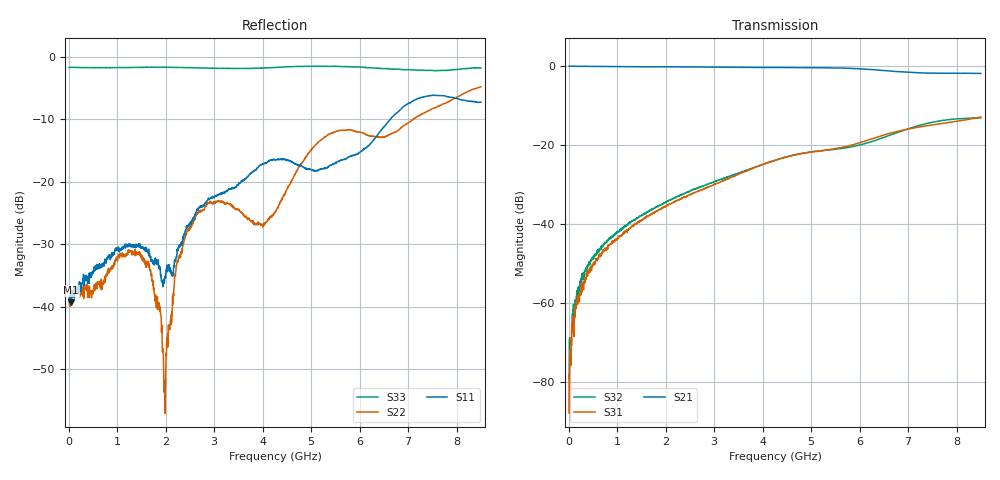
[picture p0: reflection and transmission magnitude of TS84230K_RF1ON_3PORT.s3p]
! Created with skrf (http://scikit-rf.org).
# Hz S RI R 50.0
!freq ReS11 ImS11 ReS12 ImS12 ReS13 ImS13
! ReS21 ImS21 ReS22 ImS22 ReS23 ImS23
! ReS31 ImS31 ReS32 ImS32 ReS33 ImS33
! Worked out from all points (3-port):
!   1601 points, 10 MHz to 8.5 GHz, reference 50 ohm
!   strongest paths, dB at 10 MHz, 2.132 GHz, 4.255 GHz, 6.378 GHz, 8.5 GHz:
!     S21: -0.1, -0.3, -0.4, -1.1, -1.9
!     S31: -78.0, -34.7, -23.9, -18.0, -12.9
!     S32: -78.9, -33.6, -23.9, -18.6, -13.2
!   lowest |S11| = -39.3 dB at 52.45 MHz (marker M1), VSWR 1.02, Z = 51.1 + j0.102 ohm
!   |S11| at or under -10 dB: start of sweep to 6.634 GHz
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1e7  0.0116 -0.00141  0.9876 -0.00478  7.86e-05 0.000117
     0.9871 -0.00438  0.0125 -0.0024  -0.00026 0.000218
     8.36e-05 -9.46e-05  6.4e-05 9.4e-05  -0.8229 0.00425
5.245e7  0.0108 0.000997  0.9878 -0.0159  8.61e-05 0.000302
         0.9874 -0.0161  0.0117 0.000824  0.000179 0.000622
         -4.43e-06 0.000366  5.25e-05 0.000337  -0.8235 0.017
4.504188e8  0.0169 0.00671  0.9736 -0.133  5.8e-05 0.00274
            0.9727 -0.1332  0.00984 0.00822  6.64e-05 0.00338
            -9.58e-05 0.00291  0.000224 0.0034  -0.8048 0.1536
1.469219e9  0.0287 0.0142  0.8834 -0.4065  -0.00236 0.0104
            0.883 -0.4055  0.0039 0.0272  7.83e-05 0.0124
            -0.00233 0.0105  8.87e-05 0.0126  -0.6805 0.461
1.973312e9  0.0111 -0.0109  0.8135 -0.5295  -0.00351 0.016
            0.8141 -0.5289  -0.00181 0.00102  0.000806 0.0185
            -0.00323 0.0164  0.00119 0.0185  -0.5982 0.5705
2.228012e9  -0.00237 -0.0252  0.7706 -0.587  -0.00379 0.0194
            0.7704 -0.5865  -0.012 -0.0184  0.00226 0.0219
            -0.0036 0.0194  0.00224 0.0221  -0.552 0.6069
2.652512e9  -0.035 -0.0488  0.6895 -0.6773  -0.00385 0.0253
            0.6906 -0.6757  -0.0437 -0.037  0.00513 0.0278
            -0.00388 0.0254  0.0053 0.028  -0.4752 0.6645
4.255e9  -0.00757 -0.1503  0.2984 -0.9029  0.00947 0.0633
         0.3004 -0.9025  -0.0519 0.0229  0.0346 0.0539
         0.00956 0.0633  0.0346 0.0536  -0.0471 0.8214
5.342781e9  -0.131 0.000879  -0.0282 -0.9413  0.0409 0.0766
            -0.0269 -0.9416  -0.112 0.2089  0.0717 0.0477
            0.0408 0.0768  0.0716 0.0476  0.2805 0.7924
8.5e9  -0.3655 0.2335  -0.6931 -0.4023  0.2239 0.0293
       -0.6893 -0.4049  0.2781 0.5049  0.1823 -0.1234
       0.2231 0.0304  0.1823 -0.1227  0.7526 0.3104
